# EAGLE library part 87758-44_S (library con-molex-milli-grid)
HEADER
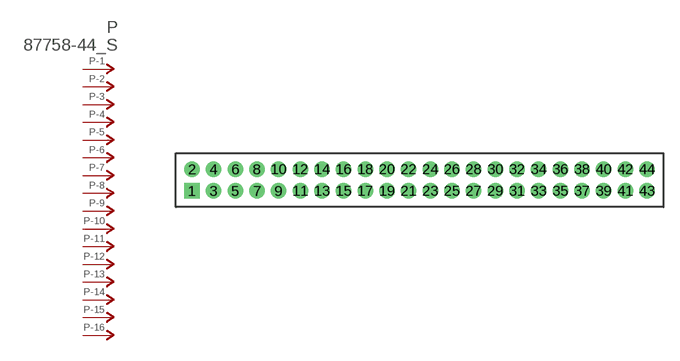
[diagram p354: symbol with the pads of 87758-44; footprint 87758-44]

Designator prefix P; gates -1=P-NV -2=P-N -3=P-N -4=P-N -5=P-N -6=P-N -7=P-N -8=P-N -9=P-N -10=P-N -11=P-N -12=P-N -13=P-N -14=P-N -15=P-N -16=P-N -17=P-N -18=P-N -19=P-N -20=P-N -21=P-N -22=P-N -23=P-N -24=P-N -25=P-N -26=P-N -27=P-N -28=P-N -29=P-N -30=P-N -31=P-N -32=P-N -33=P-N -34=P-N -35=P-N -36=P-N -37=P-N -38=P-N -39=P-N -40=P-N -41=P-N -42=P-N -43=P-N -44=P-N

## 87758-44_S  [87758-44]
1  -1:P  pas
2  -2:P  pas
3  -3:P  pas
4  -4:P  pas
5  -5:P  pas
6  -6:P  pas
7  -7:P  pas
8  -8:P  pas
9  -9:P  pas
10  -10:P  pas
11  -11:P  pas
12  -12:P  pas
13  -13:P  pas
14  -14:P  pas
15  -15:P  pas
16  -16:P  pas
17  -17:P  pas
18  -18:P  pas
19  -19:P  pas
20  -20:P  pas
21  -21:P  pas
22  -22:P  pas
23  -23:P  pas
24  -24:P  pas
25  -25:P  pas
26  -26:P  pas
27  -27:P  pas
28  -28:P  pas
29  -29:P  pas
30  -30:P  pas
31  -31:P  pas
32  -32:P  pas
33  -33:P  pas
34  -34:P  pas
35  -35:P  pas
36  -36:P  pas
37  -37:P  pas
38  -38:P  pas
39  -39:P  pas
40  -40:P  pas
41  -41:P  pas
42  -42:P  pas
43  -43:P  pas
44  -44:P  pas

## Footprint 87758-44 (pad centres in mm)
HEADER Dual Row, Vertical
drill 0.914 square: 1 -21,-1
drill 0.914: 2 -21,1; 3 -19,-1; 4 -19,1; 5 -17,-1; 6 -17,1; 7 -15,-1; 8 -15,1; 9 -13,-1; 10 -13,1; 11 -11,-1; 12 -11,1; 13 -9,-1; 14 -9,1; 15 -7,-1; 16 -7,1; 17 -5,-1; 18 -5,1; 19 -3,-1; 20 -3,1; 21 -1,-1; 22 -1,1; 23 1,-1; 24 1,1; 25 3,-1; 26 3,1; 27 5,-1; 28 5,1; 29 7,-1; 30 7,1; 31 9,-1; 32 9,1; 33 11,-1; 34 11,1; 35 13,-1; 36 13,1; 37 15,-1; 38 15,1; 39 17,-1; 40 17,1; 41 19,-1; 42 19,1; 43 21,-1; 44 21,1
